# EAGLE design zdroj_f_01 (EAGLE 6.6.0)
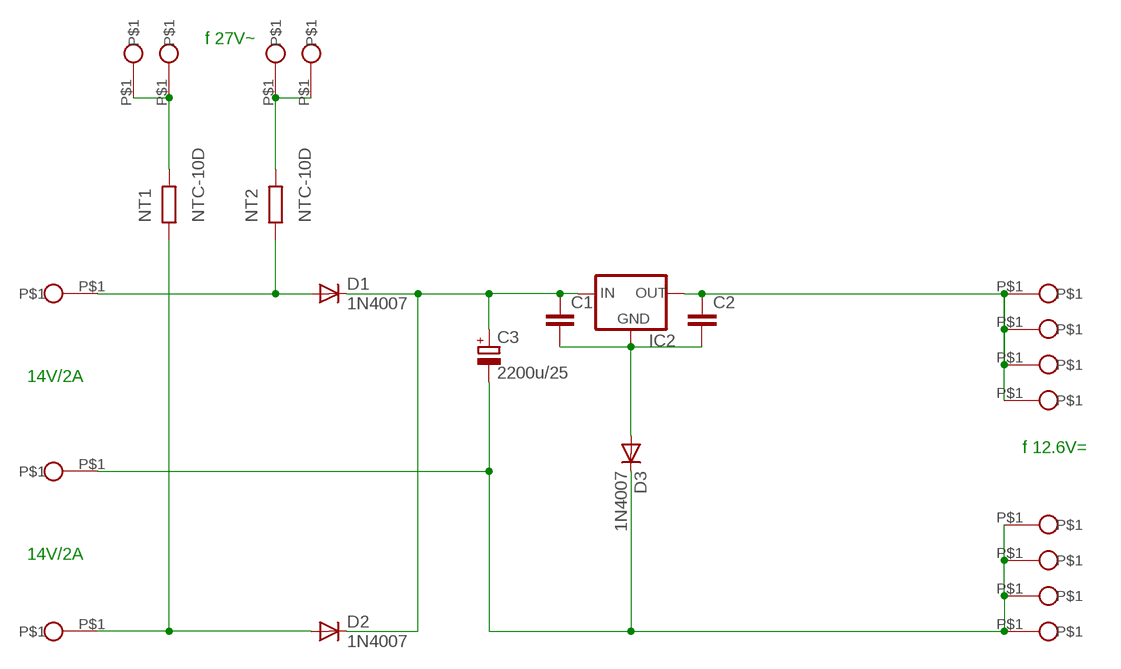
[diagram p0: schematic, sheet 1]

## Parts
C1  C-EU050-024X044  [C050-024X044]
C2  C-EU050-024X044  [C050-024X044]
C3  2200u/25  CPOL-EUE7.5-16  [E7,5-16]
D1  1N4007  1N4004  [DO41-10]
D2  1N4007  1N4004  [DO41-10]
D3  1N4007  1N4004  [DO41-10]
IC2  78XXS  [78XXS]
NT1  NTC-10D  R2WR1  [R2W]
NT2  NTC-10D  R2WR1  [R2W]
U$1  PIN  [PIN]
U$3  PIN  [PIN]
U$4  PIN  [PIN]
U$5  PIN  [PIN]
U$6  PIN  [PIN]
U$9  PIN  [PIN]
U$10  PIN  [PIN]
U$13  PIN  [PIN]
U$17  PIN  [PIN]
U$19  PIN  [PIN]
U$20  PIN  [PIN]
U$22  PIN  [PIN]
U$23  PIN  [PIN]
U$29  PIN  [PIN]
U$30  PIN  [PIN]

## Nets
GND: C3.- D3.C U$1.P$1 U$6.P$1 U$17.P$1 U$29.P$1 U$30.P$1
N$1: NT1.2 U$4.P$1 U$9.P$1
N$2: NT2.2 U$5.P$1 U$13.P$1
N$5: C1.2 C2.2 D3.A IC2.GND
N$18: D2.A NT1.1 U$19.P$1
N$19: D1.A NT2.1 U$10.P$1
N$20: C1.1 C3.+ D1.C D2.C IC2.IN
N$25: C2.1 IC2.OUT U$3.P$1 U$20.P$1 U$22.P$1 U$23.P$1

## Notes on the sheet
- f 27V~
- 14V/2A
- f 12.6V=
- 14V/2A

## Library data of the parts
C1 C2 = rcl:C-EU: CAPACITOR, European symbol
C3 = rcl:CPOL-EU: POLARIZED CAPACITOR, European symbol
D1-D3 = diode:1N4004: DIODE
IC2 = v-reg2:78XXS: VOLTAGE REGULATOR
NT1 NT2 = lampy03:R2W
U$1 U$3-U$6 U$9 U$10 U$13 U$17 U$19 U$20 U$22 U$23 U$29 U$30 = LAMPY02:PIN

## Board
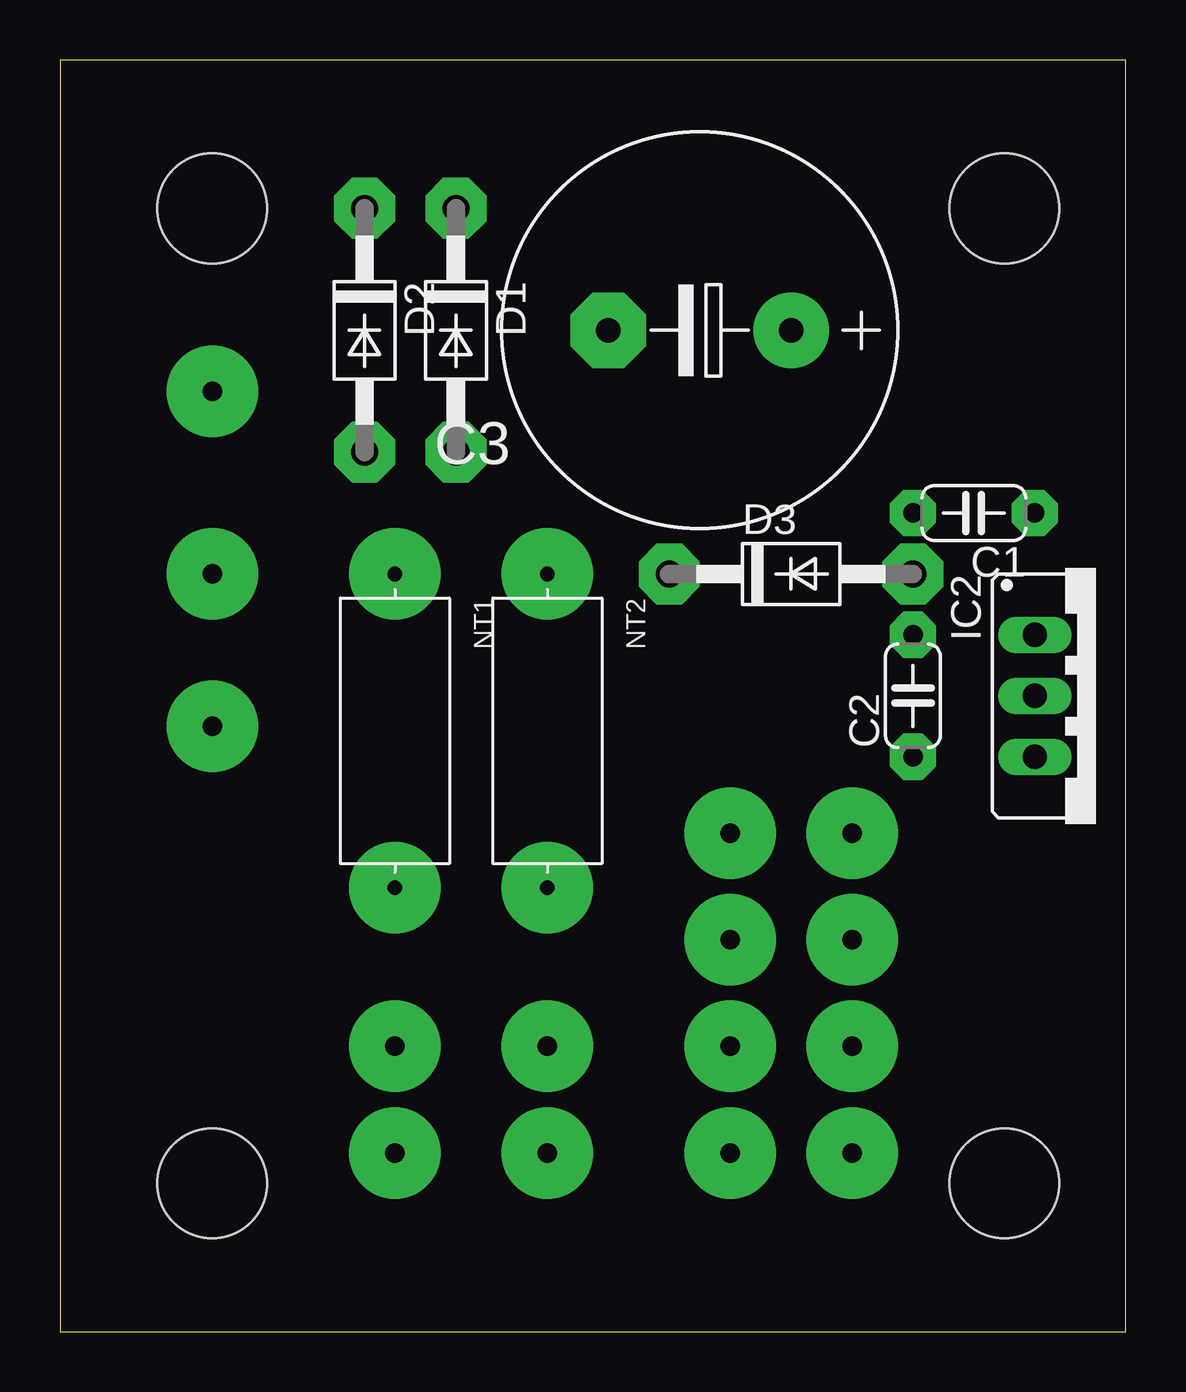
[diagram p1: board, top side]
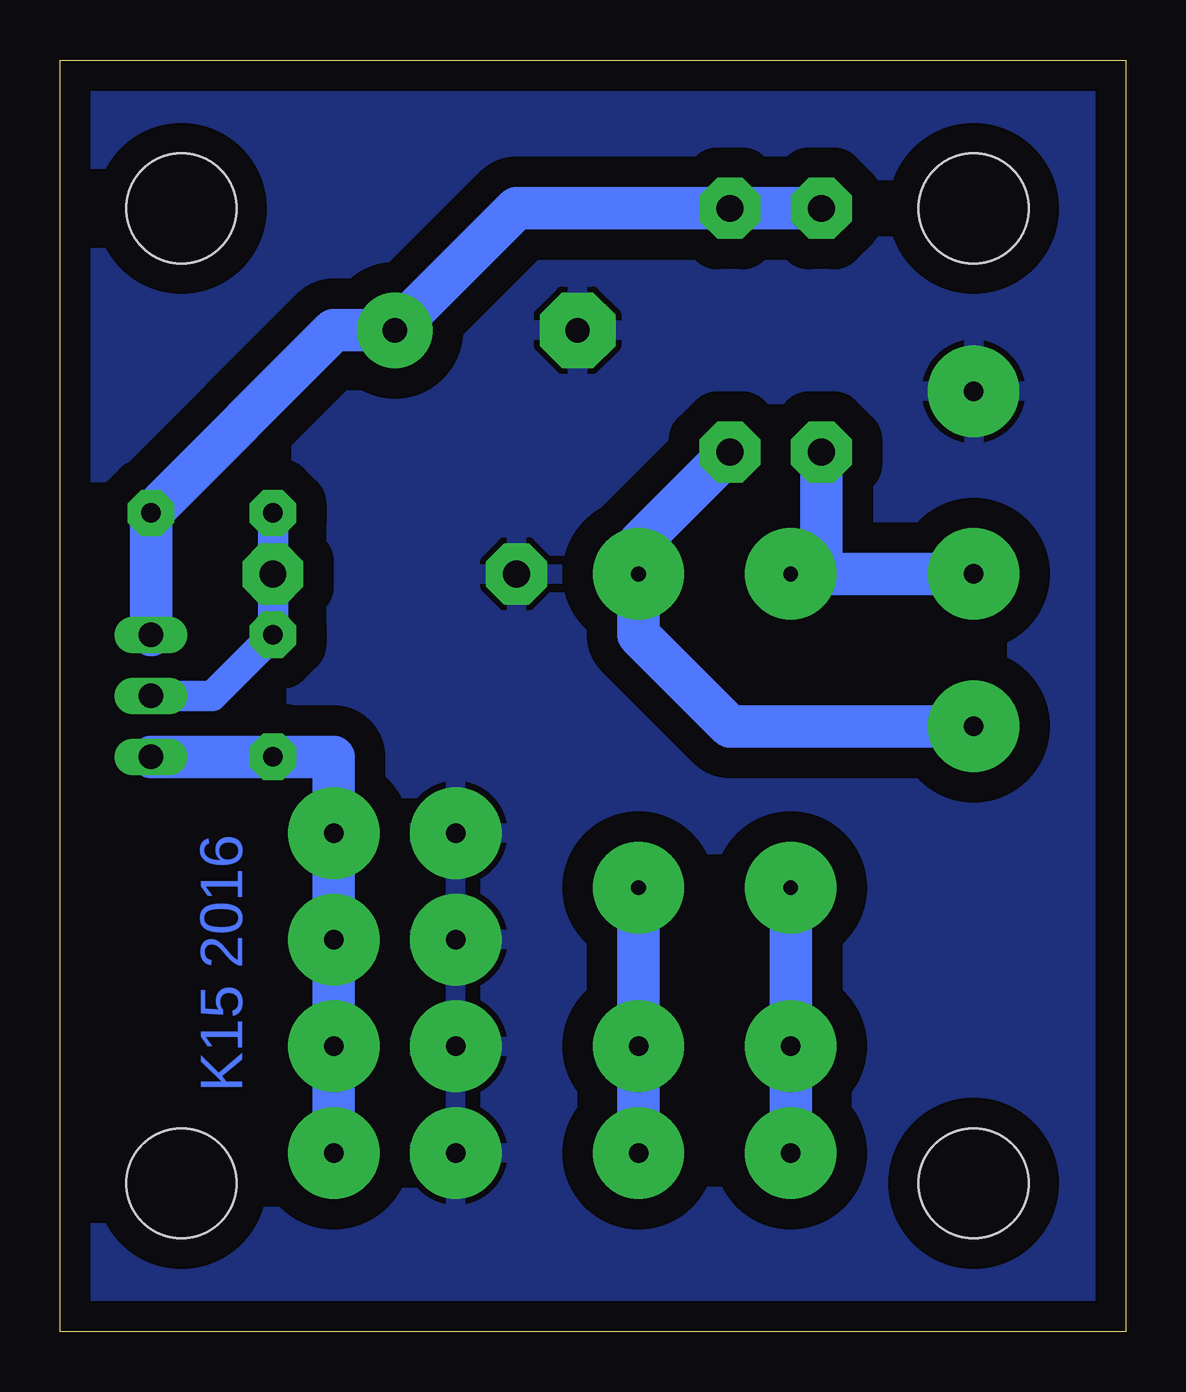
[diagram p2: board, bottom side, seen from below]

Size 44.43 x 53.01 mm. Coordinates in mm from the lower left corner, seen from the top.
Outline: 0,0 44.43,0 44.43,53.01 0,53.01 0,0
Copper layers (1*16): Top 0.035mm / dielectric 1.5mm / Bottom 0.035mm
Design rules "default": minimum track width 10mil, minimum drill 24mil, track to track 8mil, track to pad 8mil, pad to pad 8mil, via to via 8mil, smd to smd 8mil, copper to edge 40mil, drill to drill 8mil, minimum pad ring 10mil, minimum via ring 8mil, stop-mask expansion 4mil, vias tented up to drill 0mil, thermal gap 10mil
Holes 4.57 mm at 6.34,6.19 39.37,6.19 6.34,46.82 39.37,46.82

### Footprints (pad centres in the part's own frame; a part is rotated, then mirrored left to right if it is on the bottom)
C050-024X044 = drill 0.813 pad 1.93 octagon: 1 -2.54,0; 2 2.54,0
E7,5-16 = drill 1.016 pad 3.15: + -3.81,0 | drill 1.016 pad 3.15 octagon: - 3.81,0
DO41-10 = drill 1.118 pad 2.54 octagon: A 5.08,0; C -5.08,0
78XXS = drill 1.016 long: GND 0,-2.54; IN -2.54,-2.54; OUT 2.54,-2.54
R2W = drill 0.61 pad 3.81: 1 0,0; 2 13.08,0
PIN = drill 0.813 pad 3.81: P$1 0,0

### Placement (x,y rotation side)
C1  38.09,34.12 180 top
C2  35.55,26.5 90 top
C3  26.66,41.74 180 top
D1  16.5,41.74 270 top
D2  12.7,41.74 270 top
D3  30.48,31.59 0 top
IC2  43.17,26.5 270 top
NT1  13.96,31.59 270 top
NT2  20.32,31.59 270 top
U$1  27.94,16.34 0 top
U$3  33.02,20.79 0 top
U$4  13.96,11.9 270 top
U$5  20.32,11.9 90 top
U$6  27.94,20.79 0 top
U$9  13.96,7.46 0 top
U$10  6.34,25.23 0 top
U$13  20.32,7.46 180 top
U$17  27.94,7.46 0 top
U$19  6.34,31.59 0 top
U$20  33.02,7.46 0 top
U$22  33.02,11.9 0 top
U$23  33.02,16.34 0 top
U$29  27.94,11.9 0 top
U$30  6.34,39.2 0 top

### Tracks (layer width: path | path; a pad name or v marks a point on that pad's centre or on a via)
GND
  pour Bottom (isolate 1.27): 1.26,51.9 44.45,51.9 44.45,1.1 1.26,1.1
N$1
  Bottom 1.778: U$9.P$1 U$4.P$1 NT1.2
N$2
  Bottom 1.778: NT2.2 U$5.P$1 U$13.P$1
N$5
  Bottom 1.27: IC2.GND 38.09,26.5 C2.2 C1.2 D3.A
N$18
  Bottom 1.778: U$19.P$1 12.7,31.59 | D2.A 12.7,31.59 | NT1.1 12.7,31.59
N$19
  Bottom 1.778: U$10.P$1 16.5,25.23 20.32,29.05 NT2.1 20.32,32.85 D1.A
N$20
  Bottom 1.778: D2.C D1.C 25.39,46.82 C3.+ 33.02,41.74 C1.1 IC2.IN
N$25
  Bottom 1.778: U$20.P$1 U$22.P$1 U$23.P$1 U$3.P$1 33.02,23.96 C2.1 IC2.OUT

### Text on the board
Bottom: K15 2016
